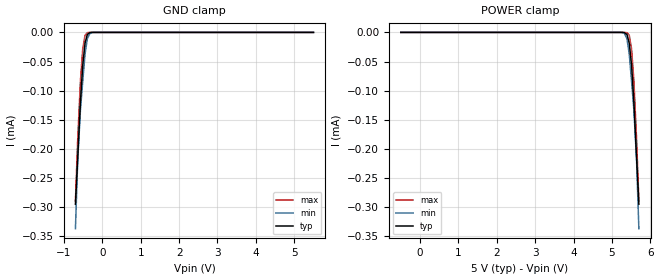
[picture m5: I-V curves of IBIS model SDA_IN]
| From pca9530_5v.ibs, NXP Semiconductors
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[Model]   SDA_IN
Model_type Input
Vinh=3.5
Vinl=1.5
C_comp   4p   3.8p   4.2p
[Temperature Range] 27   85   -40
[Voltage Range]   5   4.5   5.5
[GND Clamp]
-700mV    -295uA     -337uA     -289.5uA
-640mV    -215uA     -219.5uA   -182.9uA
-570mV    -119.6uA   -133.4uA   -83.31uA
-510mV    -56.75uA   -84.45uA   -28.37uA
-450mV    -18.67uA   -37.44uA   -5.001uA
-390mV    -3.609uA   -10.88uA   -463.2nA
-320mV    -300.6nA   -1.419uA   -19.35nA
-140mV    -201.5pA   -1.893nA   -3.612pA
5.5V      13.38pA    37.84pA    11.03pA
[POWER Clamp]
-500mV    13.38pA    37.84pA    11.03pA
5.14V     -201.5pA   -1.893nA   -3.612pA
5.32V     -300.6nA   -1.419uA   -19.35nA
5.39V     -3.609uA   -10.88uA   -463.2nA
5.45V     -18.67uA   -37.44uA   -5.001uA
5.51V     -56.75uA   -84.45uA   -28.37uA
5.57V     -119.6uA   -133.4uA   -83.31uA
5.64V     -215uA     -219.5uA   -182.9uA
5.7V      -295uA     -337uA     -289.5uA
